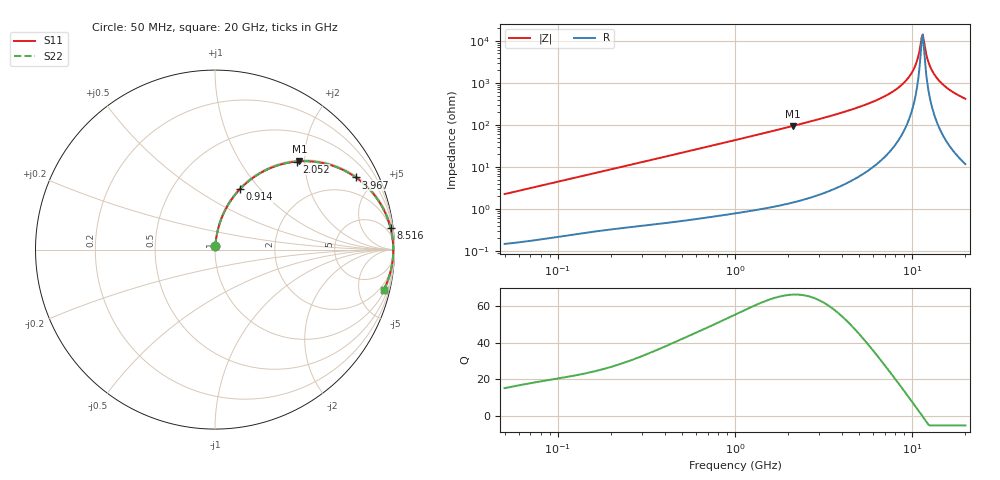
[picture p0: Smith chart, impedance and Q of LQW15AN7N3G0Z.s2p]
!Murata Part Number: LQW15AN7N3G0Z
!These Parameters are Measured in Series Mode Connection
!  o--[Z]--o
!Port1  Port2
!  o-------o
!Freq. Start=50[MHz] Stop=20[GHz], 401[Steps]
# Hz S RI R 50
!Freq.(Hz) S11(Real) S11(Imag) S21(Real) S21(Imag) S12(Real) S12(Imag) S22(Real) S22(Imag)
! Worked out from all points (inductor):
!   401 points, 50 MHz to 20 GHz, reference 50 ohm
!   read as one part in series: L = 7.18 nH near 51.52 MHz
!   highest Q = 66.1 at 2.115 GHz (marker M1), where L = 7.08 nH
!   self-resonance near 11.32 GHz
!   S11 on the Smith chart (normalised r, x): 50 MHz: 1.00, +0.05; 914 MHz: 1.01, +0.79; 2.052 GHz: 1.03, +1.82; 3.967 GHz: 1.07, +3.87; 8.516 GHz: 2, +16; 20 GHz: 1.23, -8.36
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5e7  0.00199 0.0226  0.998 -0.0226  0.998 -0.0226  0.00199 0.0226
1.364002e8  0.00627 0.06  0.9937 -0.06  0.9937 -0.06  0.00627 0.06
3.721004e8  0.0298 0.1568  0.9702 -0.1568  0.9702 -0.1568  0.0298 0.1568
9.140482e8  0.1409 0.3387  0.8591 -0.3387  0.8591 -0.3387  0.1409 0.3387
1e9  0.1635 0.3609  0.8365 -0.3609  0.8365 -0.3609  0.1635 0.3609
2.05233e9  0.4544 0.4904  0.5456 -0.4904  0.5456 -0.4904  0.4544 0.4904
2.114743e9  0.47 0.4916  0.53 -0.4916  0.53 -0.4916  0.47 0.4916
2.728004e9  0.605 0.4812  0.395 -0.4812  0.395 -0.4812  0.605 0.4812
3.967106e9  0.7849 0.4019  0.2151 -0.4019  0.2151 -0.4019  0.7849 0.4019
5.683258e9  0.9068 0.2781  0.0932 -0.2781  0.0932 -0.2781  0.9068 0.2781
7.442007e9  0.9616 0.1727  0.0384 -0.1727  0.0384 -0.1727  0.9616 0.1727
8.516016e9  0.9784 0.1188  0.0216 -0.1188  0.0216 -0.1188  0.9784 0.1188
9.457416e9  0.987 0.0768  0.013 -0.0768  0.013 -0.0768  0.987 0.0768
1.019291e10  0.9908 0.0467  0.00918 -0.0467  0.00918 -0.0467  0.9908 0.0467
1.066139e10  0.9922 0.0287  0.00776 -0.0287  0.00776 -0.0287  0.9922 0.0287
1.115139e10  0.993 0.0106  0.00701 -0.0106  0.00701 -0.0106  0.993 0.0106
1.149051e10  0.9931 -0.00138  0.00688 0.00138  0.00688 0.00138  0.9931 -0.00138
1.166392e10  0.9931 -0.0074  0.00692 0.0074  0.00692 0.0074  0.9931 -0.0074
1.257102e10  0.9918 -0.0375  0.00824 0.0375  0.00824 0.0375  0.9918 -0.0375
1.375312e10  0.9877 -0.0736  0.0123 0.0736  0.0123 0.0736  0.9877 -0.0736
1.621653e10  0.9732 -0.1398  0.0268 0.1398  0.0268 0.1398  0.9732 -0.1398
2e10  0.9403 -0.2233  0.0597 0.2233  0.0597 0.2233  0.9403 -0.2233
